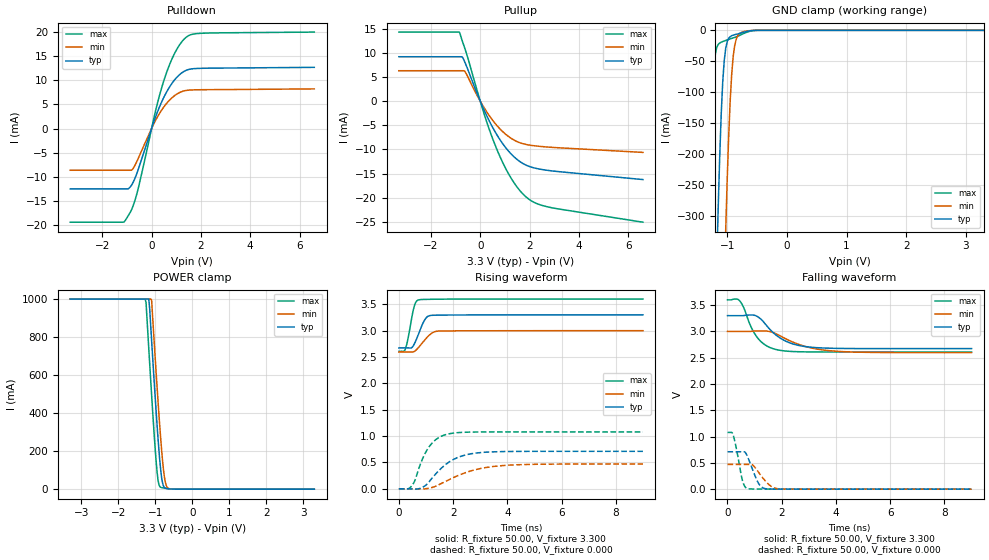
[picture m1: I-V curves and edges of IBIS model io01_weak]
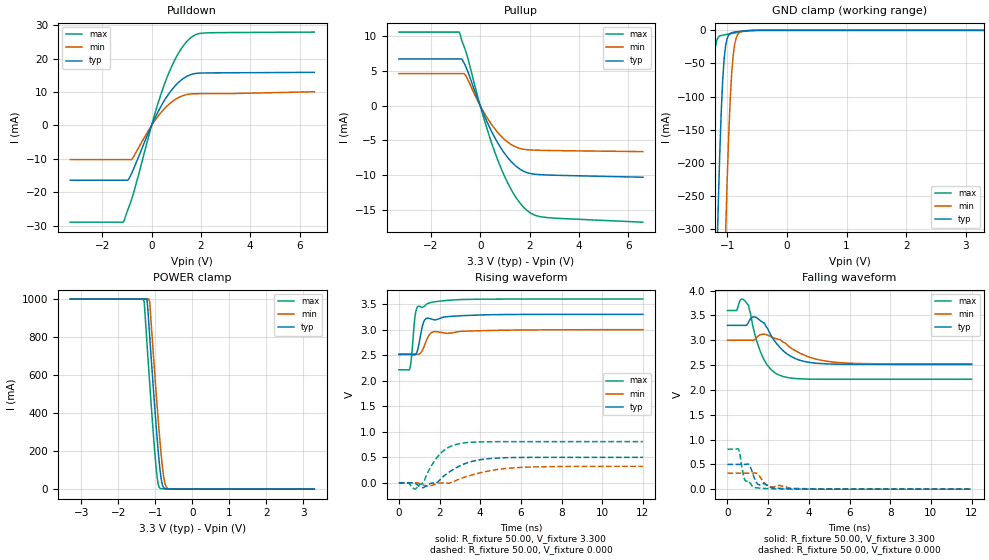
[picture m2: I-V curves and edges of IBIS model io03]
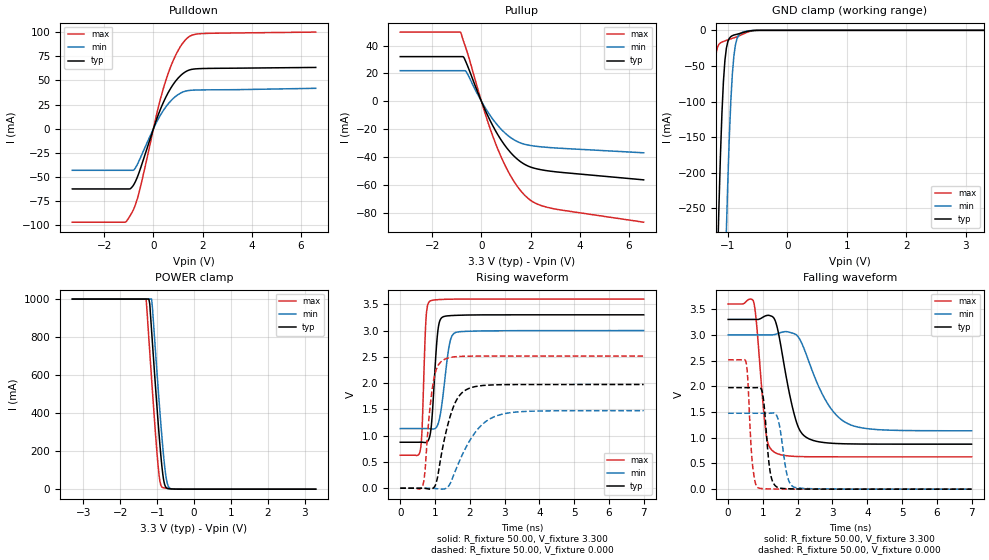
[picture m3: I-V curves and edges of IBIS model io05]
[IBIS Ver]   3.2
[File name]   rx63n_176lfbga.ibs
[File Rev]   1.00
[Date]   May 21, 2013
[Source]   From silicon level SPICE model at
   Renesas Electronics Corporation
[Notes]
|   Renesas Microcomputer RX631/RX63N Group
|   RX631/RX63N 176pin LFBGA
|   VCCQ : 3.30V
|(1) This IBIS file checked the format with ibischk5.
|   Format Error and Warning are 0.
|(2) Temperature described Tj.
|   Tj[deg]
|   Typical   45.0
|   Minimum   105.0
|   Maximum   -40.0
|(3) History
|   Rev 0.50  2012.09.10
|   New creation by Renesas Electronics Corporation
|   Rev 1.00  2013.05.21
|   Only change of revision number.
|   by Renesas Electronics Corporation
[Disclaimer]
   This information is for modeling purposes only,
   and is not guaranteed.
[Copyright]   Copyright 2012, Renesas Electronics Corporation ,
   All Rights Reserved
[Component]   rx63n_176lfbga
[Manufacturer]  Renesas Electronics Corporation
[Package]
|   typ   min   max
R_pkg   461m   461m   461m
L_pkg   3.1nH   3.1nH   3.1nH
C_pkg   0.46pF   0.46pF   0.46pF
[Pin] signal_name   model_name
A1   AVSS0   GND
A2   AVCC0   POWER
A3   VREFL0   GND
A4   P42   io14
A5   P46   io14
A6   VCC   POWER
A7   VSS   GND
A8   P94   io07
A9   VCC   POWER
A10   P97   io07
A11   PD6   io01
A12   P60   io04
A13   P63   io04
A14   PE1   io01
A15   PE2   io01
B1   P05   io02
B2   P07   io06
B3   P40   io14
B4   P41   io14
B5   P47   io14
B6   P91   io01
B7   P92   io01
B8   PD1   io01
B9   P96   io07
B10   PD4   io01
B11   PG1   io07
B12   VSS   GND
B13   P64   io04
B14   PE0   io01
B15   PE3   io01
C1   VREFL   GND
C2   VREFH   POWER
C3   VREFH0   POWER
C4   P43   io14
C5   P45   io14
C6   P90   io01
C7   PD0   io01
C8   PD2   io01
C9   PD3   io01
C10   PG0   io07
C11   VCC   POWER
C12   P62   io04
C13   PE4   io01
C14   VSS   GND
C15   P70   io04
D1   P01   io01
D2   P02   io01
D3   P03   io02
D4   P00   io01
D5   P44   io14
D6   P93   io01
D7   P95   io07
D8   VSS   GND
D9   PD5   io01
D10   PD7   io01
D11   P61   io04
D12   PE5   io01
D13   VCC   POWER
D14   PE7   io01
D15   P65   io04
E1   PJ5   io04
E2   EMLE   input06
E3   PF5   io04
E4   VSS   GND
E12   PE6   io01
E13   PG2   io07
E14   PG3   io07
E15   P67   io06
F1   VBATT   POWER
F2   VCL   POWER
F3   PJ3   io04
F4   BSCANP   input03
F12   P66   io04
F13   PG4   io07
F14   PA0   io07
F15   VSS   GND
G1   XCIN   NC
G2   XCOUT   NC
G3   MD   io04
G4   PF4   io04
G12   PG5   io04
G13   PG6   io07
G14   PA1   io07
G15   VCC   POWER
H1   P37   io05
H2   VSS   GND
H3   RES#   input02
H4   P35   input01
H12   PA4   io07
H13   PA3   io07
H14   PA2   io07
H15   PG7   io07
J1   P36   io03
J2   VCC   POWER
J3   P34   io04
J4   PF3   io04
J12   PA5   io07
J13   VSS   GND
J14   PA7   io07
J15   PA6   io07
K1   P33   io06
K2   P32   io21
K3   PF2   io04
K4   PF1   io04
K12   PB2   io07
K13   P71   io04
K14   VCC   POWER
K15   PB0   io07
L1   P31   io21
L2   P30   io21
L3   PF0   io04
L4   P25   io04
L12   PB6   io07
L13   PB3   io07
L14   PB1   io07
L15   P72   io04
M1   P27   io07
M2   P26   io07
M3   P24   io04
M4   P86   io04
M5   P13   io18
M6   P56   io07
M7   P54   io07
M8   P53   io04
M9   P50   io07
M10   PC5   io07
M11   P81   io04
M12   P77   io04
M13   PB7   io07
M14   PB5   io07
M15   PB4   io07
N1   VCC   POWER
N2   P23   io04
N3   P22   io04
N4   P15   io06
N5   P12   io18
N6   P57   io07
N7   P55   io07
N8   VCC_USB   POWER
N9   P51   io07
N10   PC7   io07
N11   P82   io04
N12   PC3   io08
N13   PC0   io17
N14   P73   io04
N15   VSS   GND
P1   VSS   GND
P2   P17   io15
P3   P87   io04
P4   P14   io06
P5   P10   io04
P6   VCC_USB   POWER
P7   VSS_USB   GND
P8   USB1_DP   io09
P9   P52   io07
P10   P83   io04
P11   PC6   io07
P12   PC4   io07
P13   PC2   io08
P14   P75   io04
P15   VCC   POWER
R1   P21   io16
R2   P20   io16
R3   P16   io15
R4   P85   io04
R5   P11   io04
R6   USB0_DM   io09
R7   USB0_DP   io09
R8   USB1_DM   io09
R9   P84   io04
R10   VSS   GND
R11   VCC   POWER
R12   P80   io04
R13   P76   io04
R14   P74   io04
R15   PC1   io17
[Diff Pin]   inv_pin   vdiff   tdelay_typ   tdelay_min   tdelay_max
R6   R7   0.000V   0.000s   NA   NA
R8   P8   0.000V   0.000s   NA   NA
[Model Selector]   io01
io01_strong   driver strength strong
io01_weak   driver strength weak
[Model Selector]   io07
io07_strong   driver strength strong
io07_weak   driver strength weak
[Model Selector]   io08
io08_strong   driver strength strong
io08_weak   driver strength weak
[Model Selector]   io15
io15a   driver strength strong
io15b   I2C buffer 1
[Model Selector]   io16
io16a   driver strength strong
io16b   I2C buffer 2
[Model Selector]   io17
io17a_strong   driver strength strong
io17a_weak   driver strength weak
io17b   I2C buffer 3
[Model Selector]   io18
io18a   driver strength strong
io18b   I2C buffer 4
| Models and submodels in the file (27): io01_strong (I/O), io01_weak (I/O), io02 (I/O), io03 (I/O), io04 (I/O), io05 (I/O), io06 (I/O), io07_strong (I/O), io07_weak (I/O), io08_strong (I/O), io08_weak (I/O), io09 (I/O), io14 (I/O), io15a (I/O), io15b (I/O_open_drain), io16a (I/O), io16b (I/O_open_drain), io17a_strong (I/O), io17a_weak (I/O), io17b (I/O_open_drain), io18a (I/O), io18b (I/O_open_drain), io21 (I/O), input01 (Input), input02 (Input), input03 (Input), input06 (Input)
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[Model]   io01_weak
Model_type   I/O
Polarity   Non-Inverting
Enable   Active-High
Vinl  =   0.660V
Vinh  =   2.640V
Vmeas =   1.650V
Cref  =   30.00pF
| variable   typ   min   max
C_comp   5.910pF   5.910pF   5.910pF
| variable   typ   min   max
[Temperature Range]   45.000   105.000   -40.000
| variable   typ   min   max
[Voltage Range]   3.300V   3.000V   3.600V
| variable   typ   min   max
[Pullup Reference]   3.300V   3.000V   3.600V
| variable   typ   min   max
[Pulldown Reference]   0.000V   0.000V   0.000V
| variable   typ   min   max
[POWER Clamp Reference] 3.300V   3.000V   3.600V
| variable   typ   min   max
[GND Clamp Reference]   0.000V   0.000V   0.000V
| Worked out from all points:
|   slope of the pulldown table from 0 to 0.495 V, typ, clamps not added: 76.6 ohm
|   slope of the pullup table from 0 to 0.495 V, typ, clamps not added: 92.4 ohm
|   GND clamp passes 1 mA (typ) near -0.63 V on its own axis
|   POWER clamp passes 1 mA (typ) near -0.58 V on its own axis
|   rising waveform, R_fixture 50.00, V_fixture 3.300: 20-80 % time 304ps typ, 415ps min, 218ps max; typ from 2.67 V to 3.3 V
|   rising waveform, R_fixture 50.00, V_fixture 0.000: 20-80 % time 931ps typ, 1.4ns min, 586ps max; typ from 0 V to 0.711 V
|   falling waveform, R_fixture 50.00, V_fixture 3.300: 20-80 % time 880ps typ, 1.24ns min, 596ps max; typ from 3.3 V to 2.67 V
|   falling waveform, R_fixture 50.00, V_fixture 0.000: 20-80 % time 333ps typ, 446ps min, 237ps max; typ from 0.711 V to 0 V
[Pulldown]
| io01_weak Pulldown rx631_rx63n
| Thu Mar 22 17:15:49 2012
| voltage   I(typ)   I(min)   I(max)
-3.3V     -12.52mA   -8.65mA    -19.43mA
-1.15V    -12.52mA   -8.65mA    -19.43mA
-1.025V   -12.52mA   -8.65mA    -18.72mA
-800mV    -11.64mA   -8.594mA   -16.68mA
-600mV    -9.336mA   -6.851mA   -13.58mA
175mV     2.596mA    1.815mA    3.964mA
525mV     6.766mA    4.671mA    10.37mA
950mV     10.19mA    6.891mA    15.75mA
1.4V      12.07mA    7.901mA    18.93mA
1.7V      12.42mA    8.02mA     19.61mA
2.1V      12.5mA     8.057mA    19.78mA
6.6V      12.7mA     8.228mA    20.01mA
[Pullup]
| io01_weak Pullup rx631_rx63n
| Thu Mar 22 17:15:49 2012
| voltage   I(typ)   I(min)   I(max)
-3.3V     9.166mA    6.276mA    14.26mA
-850mV    9.166mA    6.276mA    14.26mA
-725mV    9.114mA    6.276mA    12.4mA
-625mV    8.067mA    6.148mA    10.91mA
175mV     -2.054mA   -1.515mA   -2.91mA
700mV     -7.168mA   -5.188mA   -10.28mA
1.025V    -9.573mA   -6.827mA   -13.86mA
1.325V    -11.3mA    -7.926mA   -16.53mA
1.95V     -13.44mA   -9.058mA   -20.2mA
2.3V      -13.95mA   -9.303mA   -21.2mA
2.9V      -14.43mA   -9.565mA   -22.05mA
6.6V      -16.23mA   -10.61mA   -25.04mA
[GND Clamp]
| io01_weak GNDClamp rx631_rx63n
| Thu Mar 22 17:15:49 2012
| voltage   I(typ)   I(min)   I(max)
-3.3V     -1A        -1A        -1A
-1.325V   -1A        -1A        -369.2mA
-1.3V     -928.6mA   -1A        -269.7mA
-1.25V    -694.8mA   -1A        -112.6mA
-1.175V   -376mA     -953.3mA   -27.44mA
-1.15V    -283.8mA   -837.7mA   -22.69mA
-1.075V   -83.42mA   -512.2mA   -18.16mA
-1.025V   -28.94mA   -323mA     -16.39mA
-925mV    -8.707mA   -71.38mA   -13.1mA
-850mV    -6.468mA   -14.65mA   -10.64mA
-675mV    -1.81mA    -1.082mA   -3.186mA
3.3V      0A         0A         0A
[POWER Clamp]
| io01_weak PWRClamp rx631_rx63n
| Thu Mar 22 17:15:49 2012
| voltage   I(typ)   I(min)   I(max)
-3.3V     1A         1A         1A
-1.275V   1A         1A         1A
-1.25V    1A         1A         982.1mA
-1.175V   1A         1A         736.6mA
-1.1V     784.3mA    995.9mA    498mA
-1V       476.2mA    683.1mA    204.7mA
-950mV    332.1mA    533mA      87.52mA
-875mV    143.3mA    321.7mA    12.76mA
-825mV    55.42mA    197.2mA    7.873mA
-750mV    8.12mA     59.94mA    5.513mA
-625mV    1.619mA    2.607mA    2.132mA
3.3V      0A         0A         0A
[Ramp]
dV/dt_r   0.427/931.58p  0.283/1.40n   0.648/585.98p
dV/dt_f   0.376/877.26p  0.242/1.24n   0.595/596.02p
R_load = 50.00ohm
[Rising Waveform]
| io01_weak Rising-High rx631_rx63n
| Thu Mar 22 17:15:49 2012
R_fixture = 50.00
V_fixture = 3.300
V_fixture_min = 3.000
V_fixture_max = 3.600
C_fixture = 0.00pF
| Time   V(typ)   V(min)   V(max)
0s        2.673V     2.596V     2.608V
235ps     2.673V     2.596V     2.648V
330ps     2.674V     2.597V     2.833V
555ps     2.734V     2.602V     3.439V
630ps     2.816V     2.63V      3.544V
735ps     2.949V     2.688V     3.585V
985ps     3.229V     2.842V     3.594V
1.225ns   3.292V     2.956V     3.596V
1.57ns    3.295V     2.995V     3.598V
9ns       3.3V       3V         3.6V
[Rising Waveform]
| io01_weak Rising-Low rx631_rx63n
| Thu Mar 22 17:15:49 2012
R_fixture = 50.00
V_fixture = 0.000
C_fixture = 0.00pF
| Time   V(typ)   V(min)   V(max)
0s        0V         0V         0V
460ps     -2mV       0V         46mV
605ps     -6mV       -3mV       175mV
825ps     16mV       -4mV       509mV
1.12ns    136mV      12mV       800mV
1.435ns   324mV      67mV       960mV
1.815ns   495mV      164mV      1.039V
2.565ns   655mV      325mV      1.075V
3.875ns   707mV      442mV      1.079V
9ns       711mV      471mV      1.079V
[Falling Waveform]
| io01_weak Falling-High rx631_rx63n
| Thu Mar 22 17:15:49 2012
R_fixture = 50.00
V_fixture = 3.300
V_fixture_min = 3.000
V_fixture_max = 3.600
C_fixture = 0.00pF
| Time   V(typ)   V(min)   V(max)
0s        3.3V       3V         3.6V
350ps     3.3V       3V         3.615V
470ps     3.3V       3V         3.569V
865ps     3.312V     3.001V     3.09V
1.05ns    3.297V     3.008V     2.919V
1.4ns     3.137V     3.008V     2.739V
1.845ns   2.909V     2.942V     2.649V
2.61ns    2.735V     2.756V     2.614V
3.79ns    2.68V      2.632V     2.608V
9ns       2.673V     2.596V     2.608V
[Falling Waveform]
| io01_weak Falling-Low rx631_rx63n
| Thu Mar 22 17:15:49 2012
R_fixture = 50.00
V_fixture = 0.000
C_fixture = 0.00pF
| Time   V(typ)   V(min)   V(max)
0s        711mV      471mV      1.079V
205ps     711mV      471mV      1.037V
545ps     711mV      471mV      179mV
635ps     707mV      471mV      56mV
740ps     618mV      471mV      11mV
920ps     380mV      462mV      3mV
1.13ns    125mV      333mV      2mV
1.405ns   9mV        151mV      1mV
1.935ns   2mV        5mV        0V
9ns       0V         0V         0V
[Model]   io03
Model_type   I/O
Polarity   Non-Inverting
Enable   Active-High
Vinl  =   0.660V
Vinh  =   2.640V
Vmeas =   1.650V
Cref  =   30.00pF
| variable   typ   min   max
C_comp   4.970pF   4.970pF   4.970pF
| variable   typ   min   max
[Temperature Range]   45.000   105.000   -40.000
| variable   typ   min   max
[Voltage Range]   3.300V   3.000V   3.600V
| variable   typ   min   max
[Pullup Reference]   3.300V   3.000V   3.600V
| variable   typ   min   max
[Pulldown Reference]   0.000V   0.000V   0.000V
| variable   typ   min   max
[POWER Clamp Reference] 3.300V   3.000V   3.600V
| variable   typ   min   max
[GND Clamp Reference]   0.000V   0.000V   0.000V
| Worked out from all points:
|   slope of the pulldown table from 0 to 0.495 V, typ, clamps not added: 68.9 ohm
|   slope of the pullup table from 0 to 0.495 V, typ, clamps not added: 125 ohm
|   GND clamp passes 1 mA (typ) near -0.73 V on its own axis
|   POWER clamp passes 1 mA (typ) near -0.68 V on its own axis
|   rising waveform, R_fixture 50.00, V_fixture 3.300: 20-80 % time 250ps typ, 321ps min, 190ps max; typ from 2.51 V to 3.3 V
|   rising waveform, R_fixture 50.00, V_fixture 0.000: 20-80 % time 1.31ns typ, 1.89ns min, 877ps max; typ from 0 V to 0.499 V
|   falling waveform, R_fixture 50.00, V_fixture 3.300: 20-80 % time 1.06ns typ, 1.44ns min, 744ps max; typ from 3.3 V to 2.51 V
|   falling waveform, R_fixture 50.00, V_fixture 0.000: 20-80 % time 325ps typ, 403ps min, 271ps max; typ from 0.499 V to 0 V
[Pulldown]
| io03 Pulldown rx631_rx63n
| Thu Mar 22 17:15:49 2012
| voltage   I(typ)   I(min)   I(max)
-3.3V     -16.41mA   -10.24mA   -28.98mA
-1.15V    -16.41mA   -10.24mA   -28.98mA
-950mV    -16.26mA   -10.24mA   -24.98mA
-775mV    -13.8mA    -9.865mA   -21.27mA
100mV     1.632mA    1.118mA    2.657mA
525mV     7.544mA    5.064mA    12.43mA
800mV     10.5mA     6.935mA    17.45mA
1.075V    12.77mA    8.279mA    21.46mA
1.6V      15.26mA    9.436mA    26.34mA
1.85V     15.63mA    9.509mA    27.37mA
2.2V      15.73mA    9.534mA    27.72mA
6.6V      15.91mA    10.09mA    27.97mA
[Pullup]
| io03 Pullup rx631_rx63n
| Thu Mar 22 17:15:49 2012
| voltage   I(typ)   I(min)   I(max)
-3.3V     6.712mA    4.6mA      10.58mA
-850mV    6.712mA    4.6mA      10.58mA
-750mV    6.712mA    4.6mA      9.37mA
-600mV    5.722mA    4.374mA    7.966mA
150mV     -1.303mA   -968uA     -1.858mA
700mV     -5.288mA   -3.817mA   -7.715mA
1.3V      -8.205mA   -5.688mA   -12.35mA
1.6V      -9.105mA   -6.154mA   -13.95mA
1.925V    -9.669mA   -6.351mA   -15.16mA
2.25V     -9.879mA   -6.41mA    -15.81mA
2.7V      -9.976mA   -6.451mA   -16.1mA
6.6V      -10.3mA    -6.617mA   -16.77mA
[GND Clamp]
| io03 GNDClamp rx631_rx63n
| Thu Mar 22 17:15:49 2012
| voltage   I(typ)   I(min)   I(max)
-3.3V     -1A        -1A        -1A
-1.325V   -984.6mA   -1A        -343mA
-1.225V   -545.9mA   -1A        -51.66mA
-1.175V   -350.6mA   -894.5mA   -14.69mA
-1.15V    -263.6mA   -785.8mA   -10.32mA
-1.125V   -186.6mA   -680mA     -8.582mA
-1.075V   -73.84mA   -479.8mA   -7.226mA
-1.025V   -22.04mA   -301.7mA   -6.404mA
-975mV    -7.162mA   -158.6mA   -5.611mA
-925mV    -3.609mA   -64.96mA   -4.78mA
-800mV    -1.61mA    -3.681mA   -2.675mA
3.3V      0A         0A         0A
[POWER Clamp]
| io03 PWRClamp rx631_rx63n
| Thu Mar 22 17:15:49 2012
| voltage   I(typ)   I(min)   I(max)
-3.3V     1A         1A         1A
-1.325V   1A         1A         1A
-1.3V     1A         1A         986.2mA
-1.225V   1A         1A         768.5mA
-1.15V    800.7mA    982mA      555.2mA
-975mV    328.6mA    502.4mA    107.8mA
-925mV    209mA      374.7mA    29.63mA
-875mV    106.7mA    255.4mA    5.038mA
-825mV    36.52mA    149.8mA    2.269mA
-775mV    8.064mA    68.01mA    1.837mA
-650mV    739uA      2.543mA    864uA
3.3V      0A         0A         0A
[Ramp]
dV/dt_r   0.300/1.31n   0.193/1.89n   0.484/876.03p
dV/dt_f   0.473/1.06n   0.286/1.44n   0.832/745.27p
R_load = 50.00ohm
[Rising Waveform]
| io03 Rising-High rx631_rx63n
| Thu Mar 22 17:15:49 2012
R_fixture = 50.00
V_fixture = 3.300
V_fixture_min = 3.000
V_fixture_max = 3.600
C_fixture = 0.00pF
| Time   V(typ)   V(min)   V(max)
0s        2.512V     2.523V     2.214V
540ps     2.512V     2.523V     2.241V
625ps     2.513V     2.523V     2.477V
785ps     2.507V     2.523V     3.229V
890ps     2.563V     2.52V      3.429V
1.06ns    2.875V     2.539V     3.449V
1.22ns    3.15V      2.652V     3.45V
1.53ns    3.217V     2.917V     3.528V
3.845ns   3.286V     2.978V     3.597V
12ns      3.3V       3V         3.6V
[Rising Waveform]
| io03 Rising-Low rx631_rx63n
| Thu Mar 22 17:15:49 2012
R_fixture = 50.00
V_fixture = 0.000
C_fixture = 0.00pF
| Time   V(typ)   V(min)   V(max)
0s        0V         0V         0V
465ps     0V         0V         -1mV
810ps     -12mV      1mV        -123mV
1.2ns     -96mV      -43mV      5mV
1.575ns   -11mV      -59mV      317mV
2.07ns    80mV       -4mV       584mV
3.07ns    345mV      88mV       774mV
4.09ns    457mV      205mV      802mV
5.82ns    496mV      297mV      806mV
12ns      499mV      322mV      807mV
[Falling Waveform]
| io03 Falling-High rx631_rx63n
| Thu Mar 22 17:15:49 2012
R_fixture = 50.00
V_fixture = 3.300
V_fixture_min = 3.000
V_fixture_max = 3.600
C_fixture = 0.00pF
| Time   V(typ)   V(min)   V(max)
0s        3.3V       3V         3.6V
440ps     3.3V       3V         3.601V
865ps     3.299V     3V         3.79V
1.04ns    3.368V     3V         3.687V
1.275ns   3.471V     3.002V     3.238V
1.795ns   3.351V     3.122V     2.611V
2.775ns   2.776V     2.954V     2.265V
3.79ns    2.572V     2.698V     2.22V
5.185ns   2.52V      2.562V     2.214V
12ns      2.512V     2.523V     2.214V
[Falling Waveform]
| io03 Falling-Low rx631_rx63n
| Thu Mar 22 17:15:49 2012
R_fixture = 50.00
V_fixture = 0.000
C_fixture = 0.00pF
| Time   V(typ)   V(min)   V(max)
0s        499mV      322mV      807mV
530ps     499mV      322mV      810mV
595ps     499mV      322mV      732mV
775ps     499mV      322mV      299mV
855ps     499mV      322mV      185mV
1.085ns   481mV      322mV      134mV
1.43ns    130mV      321mV      28mV
1.89ns    91mV       94mV       12mV
2.14ns    35mV       44mV       8mV
12ns      0V         0V         0V
[Model]   io05
Model_type   I/O
Polarity   Non-Inverting
Enable   Active-High
Vinl  =   0.660V
Vinh  =   2.640V
Vmeas =   1.650V
Cref  =   30.00pF
| variable   typ   min   max
C_comp   3.770pF   3.770pF   3.770pF
| variable   typ   min   max
[Temperature Range]   45.000   105.000   -40.000
| variable   typ   min   max
[Voltage Range]   3.300V   3.000V   3.600V
| variable   typ   min   max
[Pullup Reference]   3.300V   3.000V   3.600V
| variable   typ   min   max
[Pulldown Reference]   0.000V   0.000V   0.000V
| variable   typ   min   max
[POWER Clamp Reference] 3.300V   3.000V   3.600V
| variable   typ   min   max
[GND Clamp Reference]   0.000V   0.000V   0.000V
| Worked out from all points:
|   slope of the pulldown table from 0 to 0.495 V, typ, clamps not added: 15.4 ohm
|   slope of the pullup table from 0 to 0.495 V, typ, clamps not added: 26.5 ohm
|   GND clamp passes 1 mA (typ) near -0.64 V on its own axis
|   POWER clamp passes 1 mA (typ) near -0.59 V on its own axis
|   rising waveform, R_fixture 50.00, V_fixture 3.300: 20-80 % time 140ps typ, 208ps min, 90.5ps max; typ from 0.875 V to 3.3 V
|   rising waveform, R_fixture 50.00, V_fixture 0.000: 20-80 % time 428ps typ, 745ps min, 217ps max; typ from 0 V to 1.97 V
|   falling waveform, R_fixture 50.00, V_fixture 3.300: 20-80 % time 432ps typ, 781ps min, 221ps max; typ from 3.3 V to 0.875 V
|   falling waveform, R_fixture 50.00, V_fixture 0.000: 20-80 % time 154ps typ, 198ps min, 122ps max; typ from 1.97 V to 0 V
[Pulldown]
| io05_strong Pulldown rx631_rx63n
| Thu Mar 22 17:15:49 2012
| voltage   I(typ)   I(min)   I(max)
-3.3V     -62.62mA   -43.25mA   -97.14mA
-1.15V    -62.62mA   -43.25mA   -97.14mA
-1.025V   -62.62mA   -43.25mA   -93.52mA
-800mV    -58.13mA   -42.94mA   -83.32mA
-600mV    -46.6mA    -34.2mA    -67.76mA
175mV     12.96mA    9.062mA    19.78mA
525mV     33.78mA    23.32mA    51.76mA
950mV     50.91mA    34.42mA    78.65mA
1.4V      60.32mA    39.47mA    94.53mA
1.7V      62.04mA    40.07mA    97.97mA
2.1V      62.47mA    40.25mA    98.84mA
6.6V      63.56mA    41.89mA    100.3mA
[Pullup]
| io05_strong Pullup rx631_rx63n
| Thu Mar 22 17:15:49 2012
| voltage   I(typ)   I(min)   I(max)
-3.3V     32.05mA    21.95mA    49.68mA
-850mV    32.05mA    21.95mA    49.68mA
-725mV    31.77mA    21.95mA    43.08mA
-625mV    28.07mA    21.43mA    37.88mA
175mV     -7.149mA   -5.281mA   -10.11mA
700mV     -24.99mA   -18.1mA    -35.76mA
1V        -32.82mA   -23.46mA   -47.4mA
1.325V    -39.44mA   -27.7mA    -57.61mA
1.95V     -46.99mA   -31.69mA   -70.56mA
2.3V      -48.81mA   -32.55mA   -74.14mA
2.9V      -50.5mA    -33.47mA   -77.15mA
6.6V      -56.53mA   -37.08mA   -86.96mA
[GND Clamp]
| io05_strong GNDClamp rx631_rx63n
| Thu Mar 22 17:15:49 2012
| voltage   I(typ)   I(min)   I(max)
-3.3V     -1A        -1A        -1A
-1.325V   -916.3mA   -1A        -321.6mA
-1.225V   -508.3mA   -1A        -56.05mA
-1.175V   -327.1mA   -831.8mA   -23.6mA
-1.15V    -246.5mA   -730.6mA   -19.51mA
-1.075V   -71.99mA   -445.9mA   -15.62mA
-1.025V   -24.89mA   -280.5mA   -14.09mA
-975mV    -11.12mA   -147.9mA   -12.65mA
-925mV    -7.484mA   -61.53mA   -11.26mA
-850mV    -5.559mA   -12.59mA   -9.146mA
-675mV    -1.555mA   -930uA     -2.738mA
3.3V      0A         0A         0A
[POWER Clamp]
| io05_strong PWRClamp rx631_rx63n
| Thu Mar 22 17:15:49 2012
| voltage   I(typ)   I(min)   I(max)
-3.3V     1A         1A         1A
-1.3V     1A         1A         1A
-1.225V   1A         1A         792.2mA
-1.2V     974.1mA    1A         720.1mA
-1.15V    831.4mA    1A         577.8mA
-975mV    355.2mA    535.2mA    125.1mA
-925mV    233.2mA    405.8mA    41.42mA
-875mV    126.6mA    283.8mA    11.35mA
-825mV    49.1mA     174.1mA    7.014mA
-750mV    7.224mA    53.11mA    4.912mA
-625mV    1.442mA    2.321mA    1.9mA
3.3V      0A         0A         0A
[Ramp]
dV/dt_r   1.184/427.74p  0.886/744.56p  1.509/216.62p
dV/dt_f   1.455/431.05p  1.119/780.77p  1.783/220.80p
R_load = 50.00ohm
[Rising Waveform]
| io05_strong Rising-High rx631_rx63n
| Thu Mar 22 17:15:49 2012
R_fixture = 50.00
V_fixture = 3.300
V_fixture_min = 3.000
V_fixture_max = 3.600
C_fixture = 0.00pF
| Time   V(typ)   V(min)   V(max)
0s        875mV      1.135V     628mV
575ps     876mV      1.135V     718mV
630ps     875mV      1.135V     1.161V
740ps     871mV      1.136V     3.21V
855ps     1.006V     1.133V     3.56V
1.075ns   2.955V     1.203V     3.588V
1.22ns    3.258V     1.714V     3.594V
1.415ns   3.283V     2.737V     3.597V
1.605ns   3.29V      2.967V     3.599V
7ns       3.3V       3V         3.6V
[Rising Waveform]
| io05_strong Rising-Low rx631_rx63n
| Thu Mar 22 17:15:49 2012
R_fixture = 50.00
V_fixture = 0.000
C_fixture = 0.00pF
| Time   V(typ)   V(min)   V(max)
0s        0V         0V         0V
655ps     0V         0V         69mV
950ps     3mV        -2mV       2.017V
1.065ns   184mV      -10mV      2.306V
1.25ns    871mV      -15mV      2.444V
1.485ns   1.469V     161mV      2.493V
1.715ns   1.774V     534mV      2.508V
2.205ns   1.94V      1.105V     2.514V
2.7ns     1.967V     1.36V      2.515V
7ns       1.974V     1.476V     2.515V
[Falling Waveform]
| io05_strong Falling-High rx631_rx63n
| Thu Mar 22 17:15:49 2012
R_fixture = 50.00
V_fixture = 3.300
V_fixture_min = 3.000
V_fixture_max = 3.600
C_fixture = 0.00pF
| Time   V(typ)   V(min)   V(max)
0s        3.3V       3V         3.6V
730ps     3.3V       3V         3.647V
815ps     3.299V     3V         3.228V
1.085ns   3.372V     3V         1.103V
1.325ns   3.315V     3.005V     721mV
1.915ns   1.417V     3.019V     637mV
2.255ns   1.003V     2.603V     631mV
2.855ns   899mV      1.669V     629mV
3.44ns    881mV      1.274V     628mV
7ns       875mV      1.135V     628mV
[Falling Waveform]
| io05_strong Falling-Low rx631_rx63n
| Thu Mar 22 17:15:49 2012
R_fixture = 50.00
V_fixture = 0.000
C_fixture = 0.00pF
| Time   V(typ)   V(min)   V(max)
0s        1.974V     1.476V     2.515V
515ps     1.974V     1.476V     2.465V
690ps     1.973V     1.476V     547mV
855ps     1.976V     1.476V     29mV
1.01ns    1.773V     1.476V     9mV
1.215ns   310mV      1.477V     4mV
1.405ns   40mV       1.419V     2mV
1.695ns   9mV        274mV      1mV
1.885ns   5mV        42mV       0V
7ns       0V         0V         0V
